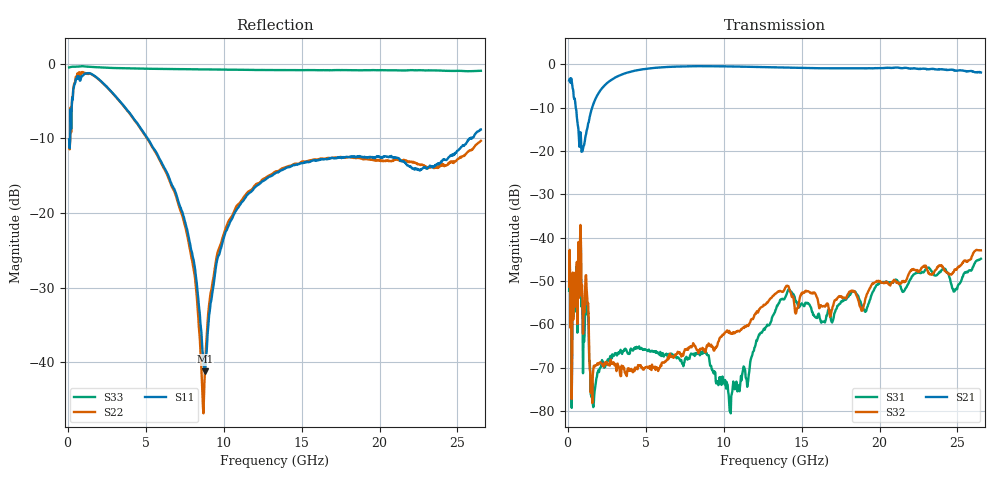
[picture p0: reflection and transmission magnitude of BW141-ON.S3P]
!  3-Port S-parameters saved by WinCal
! VAR MeasName=S-Parameters (CALIBRATED_DATA) read from VNA (N5242A)
! VAR MeasDate=2014-8-25 14:20:19
! VAR NAME=1
! VAR FILENAME=1.S3P
! VAR DATE=2014-8-25 14:20:19
! VAR PHYS_PORTS=1,2,3
# Hz S MA R 50
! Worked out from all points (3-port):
!   801 points, 100 MHz to 26.5 GHz, reference 50 ohm
!   strongest paths, dB at 100 MHz, 6.7 GHz, 13.3 GHz, 19.9 GHz, 26.5 GHz:
!     S21: -3.8, -0.6, -0.7, -0.9, -1.9
!     S32: -51.3, -67.3, -52.9, -50.1, -42.9
!     S31: -52.3, -66.8, -57.1, -50.8, -44.9
!   lowest |S11| = -41.2 dB at 8.812 GHz (marker M1), VSWR 1.02, Z = 50.8 - j0.438 ohm
!   |S11| at or under -10 dB: start of sweep to 166 MHz; 5.14 GHz to 25.77 GHz (20.63 GHz wide, 133 % of centre); 25.8204 GHz to 25.84704 GHz (26.63 MHz wide, 0.103 % of centre)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
1e8  0.3123 -164.2  0.6463 -7.5  0.002462 -78.3
     0.648 -7.5  0.3107 -165.0  0.002759 -78.1
     0.002439 -78.2  0.002727 -78.0  0.9463 -179.8
3.31e8  0.575 -152.1  0.5237 -33.5  0.003629 -22.3
        0.5262 -33.3  0.5794 -151.9  0.003943 -21.4
        0.003647 -21.4  0.003967 -21.3  0.9567 179.5
7.93e8  0.7697 -179.7  0.1422 -10.4  0.007269 -78.8
        0.1436 -10.1  0.8435 177.7  0.008176 -64.7
        0.007385 -76.5  0.008167 -65.0  0.9602 178.1
1.618e9  0.845 155.2  0.3305 54.1  0.0001248 67.9
         0.332 53.9  0.8419 152.5  0.0002611 -111.2
         0.0001219 65.2  0.0002584 -104.8  0.9524 175.5
6.898e9  0.1399 74.2  0.9374 -20.3  0.0004216 37.8
         0.9367 -20.4  0.1348 69.5  0.0004516 -161.7
         0.0004249 37.9  0.0004496 -161.6  0.9227 164.9
8.812e9  0.00872 -29.7  0.9469 -37.3  0.0004792 21.0
         0.9472 -37.3  0.008777 -175.6  0.0004778 -165.5
         0.0004799 20.8  0.0004917 -166.0  0.9178 161.1
1.0429e10  0.08772 -123.5  0.9386 -50.1  9.433e-05 -13.1
           0.9402 -50.1  0.09203 -148.1  0.0007733 -165.8
           0.000103 -28.4  0.0007871 -165.5  0.9142 157.8
1.33e10  0.1838 -141.9  0.9139 -70.6  0.001379 -154.7
         0.9174 -70.4  0.1889 -170.6  0.002213 -178.0
         0.001395 -153.8  0.002254 -177.0  0.9078 152.1
1.8877e10  0.237 -162.3  0.8918 -106.9  0.001637 133.6
           0.8968 -106.7  0.2307 140.4  0.001429 143.4
           0.001622 134.1  0.001436 143.5  0.9052 140.3
2.65e10  0.3635 -137.2  0.78 -169.8  0.005506 138.9
         0.8027 -171.4  0.3049 -26.4  0.007121 92.3
         0.005716 140.8  0.007145 95.8  0.8984 122.8
